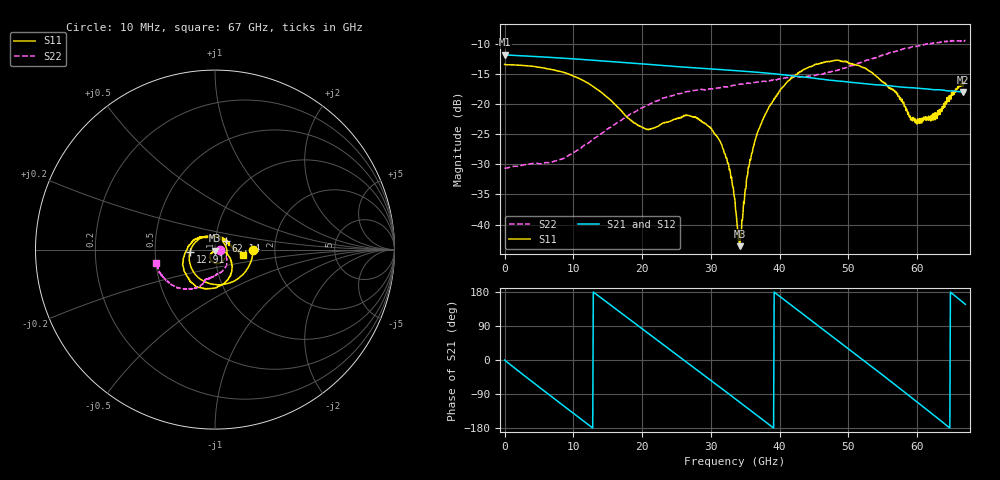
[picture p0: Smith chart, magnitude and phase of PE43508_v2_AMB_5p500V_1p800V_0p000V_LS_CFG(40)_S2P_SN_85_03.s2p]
!Keysight Technologies,N5227A,US51270237,A.10.43.00
!Date: Wednesday, August 22, 2018 17:10:44
!Correction: S11(Full 2 Port(1,3))
!S31(Full 2 Port(1,3))
!S13(Full 2 Port(1,3))
!S33(Full 2 Port(1,3))
!S2P File: Measurements: S11, S31, S13, S33:
# Hz S  dB  R 50
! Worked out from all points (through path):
!   801 points, 10 MHz to 67 GHz, reference 50 ohm
!   highest |S21| = -11.84 dB at 10 MHz (marker M1); lowest = -18.0 dB at 66.67 GHz (marker M2)
!   group delay of S21, straight-line fit = 38.4 ps
!   lowest |S11| = -43.6 dB at 34.17 GHz (marker M3), VSWR 1.01, Z = 50 - j0.663 ohm
!   |S11| at or under -10 dB: start of sweep to end of sweep
!   |S22| runs from -30.6 to -9.5 dB; largest |S21 - S12| = 0.0011
!   S11 on the Smith chart (normalised r, x): 10 MHz: 1.54, -0.00; 12.91 GHz: 0.76, -0.02; 62.14 GHz: 1.12, +0.11; 67 GHz: 1.36, -0.09
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1e7  -13.42 -0.4  -11.84 -0.2  -11.85 -0.2  -30.62 -0.5
5.70415e9  -14.03 -80.1  -12.20 -80.9  -12.21 -80.9  -29.79 -14.5
1.123082e10  -15.99 -152.5  -12.60 -157.6  -12.61 -157.5  -27.15 -19.5
1.290558e10  -17.11 -175.0  -12.74 179.4  -12.74 179.4  -25.79 -21.5
1.792982e10  -22.34 101.6  -13.15 110.4  -13.15 110.4  -21.96 -36.4
2.236791e10  -23.64 -2.8  -13.56 49.8  -13.56 49.8  -19.39 -54.3
2.655479e10  -21.86 -71.9  -13.92 -7.1  -13.92 -7.1  -17.93 -70.7
2.982055e10  -23.77 -109.7  -14.18 -51.5  -14.17 -51.5  -17.48 -80.7
3.224894e10  -29.02 -131.3  -14.36 -84.7  -14.36 -84.6  -17.16 -86.0
3.3505e10  -36.00 -128.5  -14.46 -102.0  -14.46 -102.0  -16.88 -89.0
3.392369e10  -41.12 -114.7  -14.49 -107.7  -14.50 -107.7  -16.76 -90.1
3.41749e10  -43.57 -88.0  -14.51 -111.1  -14.52 -111.1  -16.72 -90.1
3.559844e10  -30.02 -6.9  -14.63 -130.9  -14.64 -130.8  -16.57 -92.4
3.75244e10  -22.69 -20.8  -14.81 -157.5  -14.82 -157.5  -16.25 -95.9
4.095764e10  -16.52 -51.0  -15.21 154.7  -15.21 154.8  -15.65 -101.6
4.472582e10  -13.72 -84.7  -15.68 102.4  -15.67 102.5  -15.33 -106.5
4.975008e10  -13.07 -128.5  -16.33 33.0  -16.32 33.0  -13.96 -109.5
5.586291e10  -17.38 164.6  -16.96 -52.4  -16.95 -52.8  -11.56 -123.5
5.937989e10  -22.21 104.7  -17.31 -102.1  -17.33 -102.3  -10.50 -134.7
6.214322e10  -22.34 39.3  -17.59 -142.0  -17.60 -142.2  -9.95 -146.0
6.666505e10  -16.99 -9.7  -18.02 151.8  -18.07 151.8  -9.52 -164.9
6.7e10  -16.01 -11.5  -18.01 146.8  -18.08 146.8  -9.51 -167.1
